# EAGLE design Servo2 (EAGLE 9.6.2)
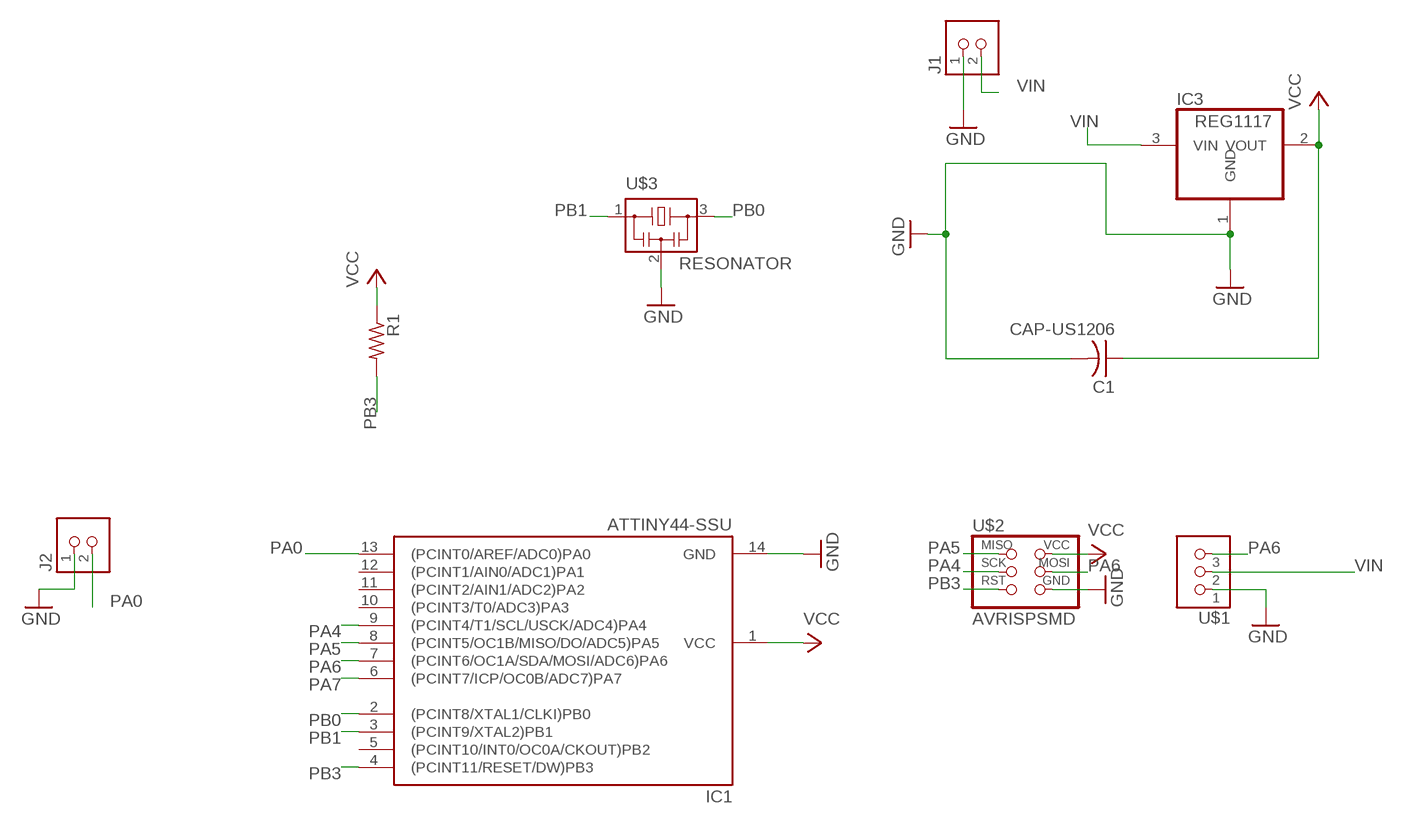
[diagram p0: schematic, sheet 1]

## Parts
C1  CAP-US1206  [C1206]
IC1  ATTINY44-SSU  [SOIC14]
IC3  REG1117  [SOT223]
J1  CONN_02_TERM-ADAFRUIT  [3.5MMTERM]
J2  CONN_02_TERM-ADAFRUIT  [3.5MMTERM]
R1  RES-US1206  [R1206]
U$1  CONN_03_TERM'-FABLAB'  [ED555DS-3DS]
U$2  AVRISPSMD  [2X03SMD]
U$3  RESONATOR  [EFOBM]

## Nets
GND: C1.2 IC1.14(GND) IC3.1(GND) J1.1 J2.1 U$1.1 U$2.6(GND) U$3.2
PA0: IC1.13((PCINT0/AREF/ADC0)PA0) J2.2
PA4: IC1.9((PCINT4/T1/SCL/USCK/ADC4)PA4) U$2.3(SCK)
PA5: IC1.8((PCINT5/OC1B/MISO/DO/ADC5)PA5) U$2.1(MISO)
PA6: IC1.7((PCINT6/OC1A/SDA/MOSI/ADC6)PA6) U$1.3 U$2.4(MOSI)
PA7: IC1.6((PCINT7/ICP/OC0B/ADC7)PA7)
PB0: IC1.2((PCINT8/XTAL1/CLKI)PB0) U$3.3
PB1: IC1.3((PCINT9/XTAL2)PB1) U$3.1
PB3: IC1.4((PCINT11/RESET/DW)PB3) R1.2 U$2.5(RST)
VCC: C1.1 IC1.1(VCC) IC3.2(VOUT) R1.1 U$2.2(VCC)
VIN: IC3.3(VIN) J1.2 U$1.2
Unconnected: IC1.5((PCINT10/INT0/OC0A/CKOUT)PB2) IC1.10((PCINT3/T0/ADC3)PA3) IC1.11((PCINT2/AIN1/ADC2)PA2) IC1.12((PCINT1/AIN0/ADC1)PA1)

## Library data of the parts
C1 = fab:CAP-US
IC1 = fab:ATTINY44
IC3 = burr-brown:REG1117: 800mA and 1A Low Dropout (LDO) Positive Regulator 1.8V, 2.5V, 2.85V, 3.3V, 5V, and Adj; MPN: REG1117; OC_FARNELL: 1097566; OC_NEWARK: 14P6981
J1 J2 = fab:CONN_02_TERM: 3.5mm terminal block, 2 positions ED555-2DS as found in the fablab inventory.
R1 = fab:RES-US: Resistor (US Symbol)
U$1 = fab:CONN_03_TERM: 3.5mm terminal block, 3 positions ED555-3DS as found in the fablab inventory. Made by Zaerc.
U$2 = fab:AVRISP
U$3 = fab:RESONATOR

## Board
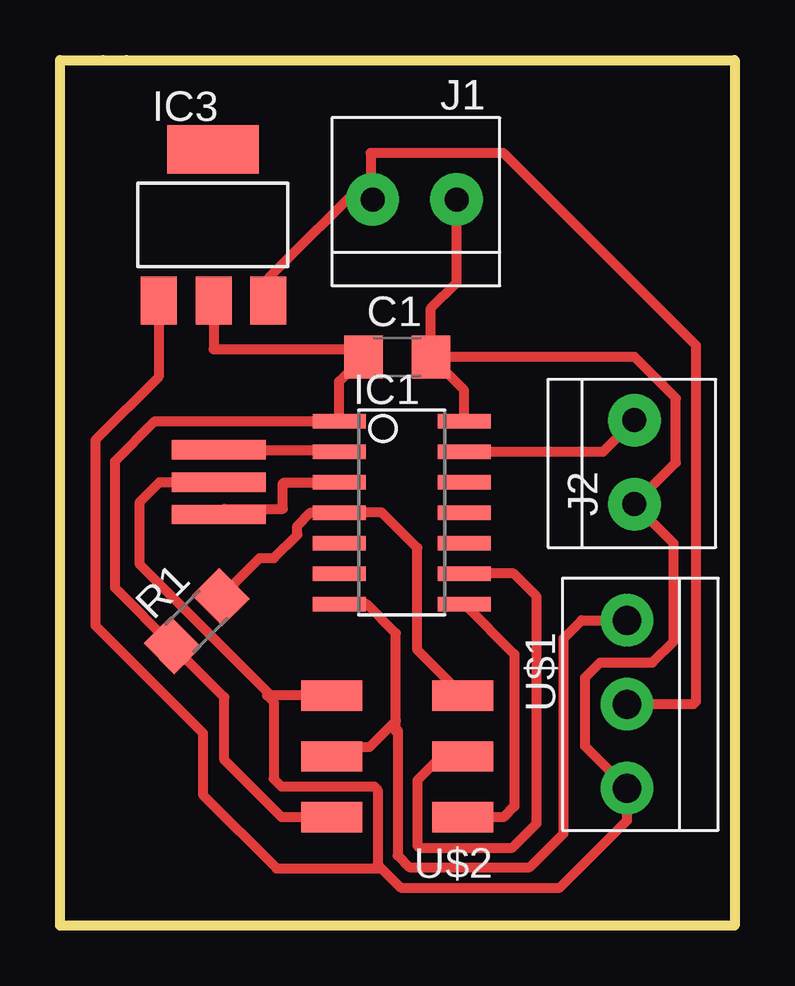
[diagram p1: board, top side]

Size 28.11 x 36.09 mm. Coordinates in mm from the lower left corner, seen from the top.
Outline: 1.79,36.09 28.11,36.09 28.11,0 0,0 0,36.08 2.76,36.08
Copper layers (1*16): Top 0.035mm / dielectric 1.5mm / Bottom 0.035mm
Design rules "default *": minimum track width 6mil, minimum drill 0.35mm, track to track 16mil, track to pad 16mil, pad to pad 16mil, via to via 16mil, smd to smd 16mil, copper to edge 40mil, drill to drill 6mil, minimum pad ring 10mil, minimum via ring 8mil, stop-mask expansion 4mil, vias tented up to drill 0mil, thermal gap 10mil

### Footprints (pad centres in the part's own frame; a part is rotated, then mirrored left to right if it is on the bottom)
C1206 = smd 1.6 x 1.8: 1 -1.4,0; 2 1.4,0
SOIC14 = smd 0.61 x 2.21: 1 -3.81,-2.603; 2 -2.54,-2.603; 3 -1.27,-2.603; 4 0,-2.603; 5 1.27,-2.603; 6 2.54,-2.603; 7 3.81,-2.603; 8 3.81,2.603; 9 2.54,2.603; 10 1.27,2.603; 11 0,2.603; 12 -1.27,2.603; 13 -2.54,2.603; 14 -3.81,2.603
SOT223 = smd 1.499 x 2.007: 1 -2.261,-3.15; 2 0.025,-3.15; 3 2.311,-3.15 | smd 3.81 x 2.007: 4 0,3.15
3.5MMTERM = drill 1 pad 2.184: 1 1.8,0; 2 -1.7,0
R1206 = smd 1.6 x 1.803: 1 -1.422,0; 2 1.422,0
ED555DS-3DS = drill 1.2 pad 2.184: 1 -3.5,0; 2 0,0; 3 3.5,0
2X03SMD = smd 2.54 x 1.27: 1 -2.54,2.54; 2 2.92,2.54; 3 -2.54,0; 4 2.92,0; 5 -2.54,-2.54; 6 2.92,-2.54
EFOBM = smd 0.8 x 3.9: 1 -1.35,0; 2 0,0; 3 1.35,0

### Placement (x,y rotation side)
C1  14.05,23.7 0 top
IC1  14.24,17.22 270 top
IC3  6.37,29.21 0 top
J1  14.72,30.27 0 top
J2  23.93,19.37 270 top
R1  5.69,12.69 45 top
U$1  23.63,9.22 90 top
U$2  14.24,7.06 180 top
U$3  6.62,18.49 90 top

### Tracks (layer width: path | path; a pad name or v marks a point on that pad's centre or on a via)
GND
  Top 0.406: IC1.14 16.84,22.32 C1.2 | U$2.6 8.79,9.6 | 8.79,9.6 8.63,9.6 8.9,9.32 8.9,6.13 9.23,5.8 13.1,5.8 13.24,5.66 13.24,2.54 13.39,2.39 | 8.79,9.6 3.33,15.05 3.33,17.67 4.15,18.49 U$3.2 | C1.2 23.95,23.7 25.66,21.99 25.66,19.3 J2.1 25.56,15.93 25.56,11.85 24.68,10.97 22.5,10.97 21.88,10.34 21.88,7.48 U$1.1 23.63,4.38 20.83,1.58 14.2,1.58 13.39,2.39 | C1.2 15.45,25.74 16.52,26.81 J1.1 | IC3.1 4.11,22.87 1.48,20.24 1.48,12.51 5.96,8.03 5.96,5.45 9.02,2.39 13.39,2.39
PA0
  Top 0.406: J2.2 22.62,19.75 IC1.13
PA4
  Top 0.406: U$2.3 15.89,7.06 14.89,6.06 14.89,3.33 14.97,3.25 18.85,3.25 19.86,4.26 19.86,13.72 18.91,14.68 IC1.9
PA5
  Top 0.406: IC1.8 18.94,11.31 18.94,4.97 18.48,4.52 U$2.1
PA6
  Top 0.406: U$2.4 11.7,7.44 12.88,7.44 13.99,8.54 | IC1.7 12.78,13.41 13.99,12.19 13.99,8.54 | 13.99,8.54 13.99,8.08 14.07,8.16 14.07,2.92 14.56,2.43 19.56,2.43 20.98,3.85 20.98,11.97 21.73,12.72 U$1.3
PB0
  Top 0.406: U$3.3 11.55,19.84 IC1.2
PB1
  Top 0.406: U$3.1 6.86,17.38 9.29,17.38 9.29,18.45 11.59,18.45 IC1.3
PB3
  Top 0.406: U$2.5 14.89,11.49 14.89,15.74 13.41,17.22 IC1.4 10.43,17.22 9.89,16.67 9.89,16.29 8.91,15.32 8.32,15.32 R1.2
VCC
  Top 0.406: U$2.2 9.24,4.52 6.85,6.9 6.85,9.52 R1.1 2.29,14.08 2.29,19.36 3.96,21.03 IC1.1 11.63,22.68 C1.1 12.33,24.03 6.4,24.03 IC3.2
VIN
  Top 0.406: 12.86,31.17 8.69,26.99 8.69,25.53 8.68,25.53 IC3.3 | 12.86,31.17 12.94,31.24 12.94,32.22 18.47,32.22 26.49,24.19 26.49,9.33 26.39,9.22 U$1.2 | 12.86,31.17 12.86,30.43 J1.2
